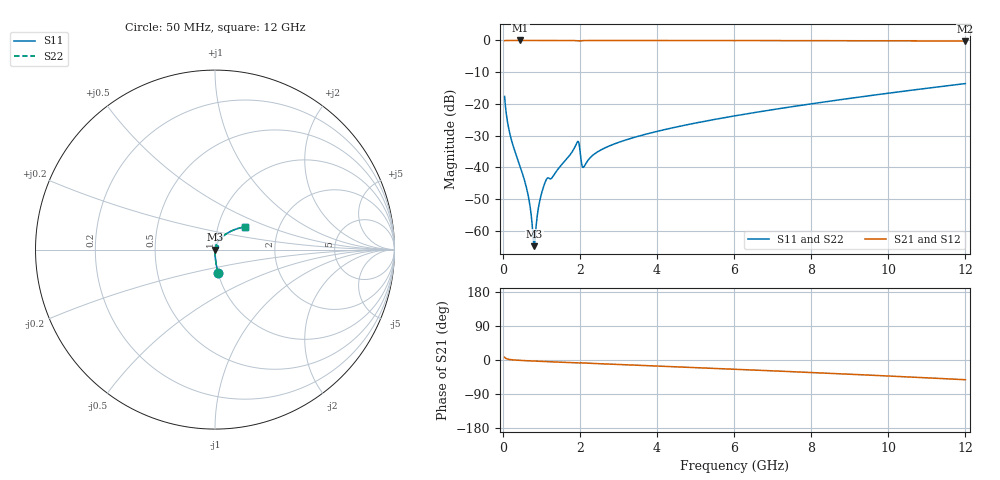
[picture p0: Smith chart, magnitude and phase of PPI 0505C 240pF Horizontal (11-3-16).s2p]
# MHz S MA R 50
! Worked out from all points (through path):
!   1601 points, 50 MHz to 12 GHz, reference 50 ohm
!   highest |S21| = 0.00 dB at 453.3 MHz (marker M1); lowest = -0.2 dB at 12 GHz (marker M2)
!   group delay of S21, straight-line fit = 12.1 ps
!   lowest |S11| = -64.9 dB at 819.3 MHz (marker M3), VSWR 1.00, Z = 50.1 + j0.00123 ohm
!   |S11| at or under -10 dB: start of sweep to end of sweep
!   |S22| runs from -64.9 to -13.6 dB; largest |S21 - S12| = 0
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50  0.1308 -82.6  0.9912 7.3  0.9912 7.3  0.1308 -82.6
199.375  0.03128 -88.3  0.9992 1.1  0.9992 1.1  0.03128 -88.3
453.3125  0.01023 -88.6  0.9995 -1.0  0.9995 -1.0  0.01023 -88.6
647.5  0.003939 -84.7  0.9995 -2.0  0.9995 -2.0  0.003939 -84.7
707.25  0.002485 -80.2  0.9994 -2.3  0.9994 -2.3  0.002485 -80.2
781.9375  0.0009296 -56.3  0.9994 -2.7  0.9994 -2.7  0.0009296 -56.3
819.2812  0.00057 1.2  0.9994 -2.9  0.9994 -2.9  0.00057 1.2
856.625  0.0009983 50.8  0.9994 -3.0  0.9994 -3.0  0.0009983 50.8
976.125  0.003247 73.8  0.9992 -3.6  0.9992 -3.6  0.003247 73.8
1132.969  0.006418 70.2  0.9982 -4.3  0.9982 -4.3  0.006418 70.2
1297.281  0.007073 72.5  0.9984 -4.9  0.9984 -4.9  0.007073 72.5
1924.656  0.02448 59.2  0.9901 -8.0  0.9901 -8.0  0.02448 59.2
1969.469  0.02475 38.5  0.9826 -7.9  0.9826 -7.9  0.02475 38.5
2044.156  0.01173 28.0  0.9903 -7.5  0.9903 -7.5  0.01173 28.0
2111.375  0.01026 57.0  0.9955 -7.9  0.9955 -7.9  0.01026 57.0
2342.906  0.01557 75.2  0.9982 -9.0  0.9982 -9.0  0.01557 75.2
2671.531  0.02047 76.2  0.9984 -10.4  0.9984 -10.4  0.02047 76.2
4038.312  0.03725 72.1  0.9979 -16.1  0.9979 -16.1  0.03725 72.1
6025  0.06475 64.4  0.9962 -24.4  0.9962 -24.4  0.06475 64.4
8019.156  0.1005 56.0  0.9928 -33.1  0.9928 -33.1  0.1005 56.0
10013.31  0.1476 47.0  0.9865 -42.3  0.9865 -42.3  0.1476 47.0
12000  0.2088 37.3  0.975 -52.1  0.975 -52.1  0.2088 37.3
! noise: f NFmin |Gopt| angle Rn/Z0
50  0.0003254  0.84  0.2894  0.0004307
1372  0.004074  0.6801  4.739  0.002459
2701  0.005777  0.5829  9.202  0.002509
4031  0.00711  0.5177  13.47  0.002544
5360  0.008699  0.4894  17.63  0.002861
6682  0.01029  0.4726  21.63  0.003205
8012  0.0119  0.4631  25.5  0.003576
9341  0.01356  0.4593  29.22  0.003982
1.067e+04  0.0153  0.4603  32.78  0.004437
1.2e+04  0.01714  0.4654  36.21  0.004956
